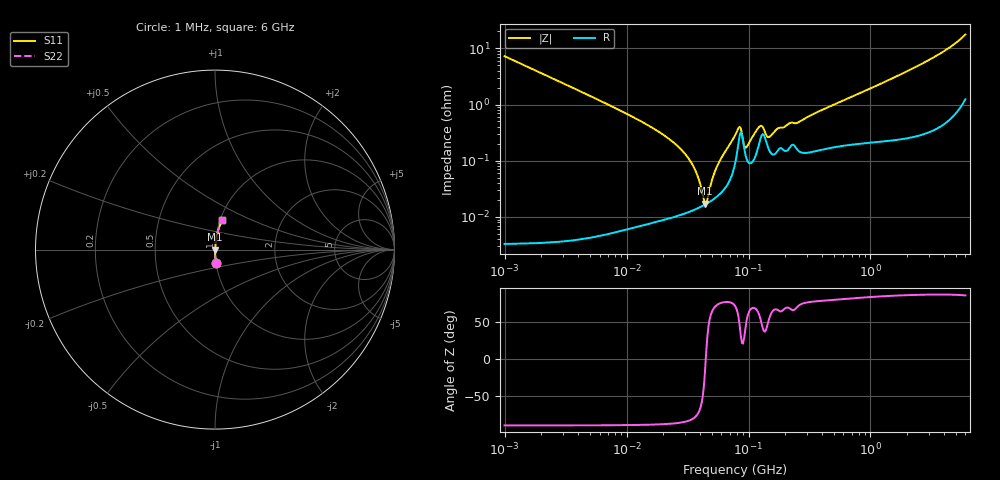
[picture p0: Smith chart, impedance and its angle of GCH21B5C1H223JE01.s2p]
!Murata Part Number: GCH21B5C1H223JE01
!These Parameters are Measured in Series Mode Connection
!Data Generated on Jun 19, 2026
!  o--ll--o
!Port1  Port2
!  o------o
!Operation Temp=25[degC], DC Bias Voltage=0[V]
!Freq. Start=1000[kHz] Stop=6[GHz] 401[Steps]
# Hz S RI R 50
!Freq.(Hz) S11(Real) S11(Imag) S21(Real) S21(Imag) S12(Real) S12(Imag) S22(Real) S22(Imag)
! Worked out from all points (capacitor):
!   401 points, 1 MHz to 6 GHz, reference 50 ohm
!   read as one part in series: C = 22 nF near 1.044 MHz
!   lowest |Z| = 17.3 mohm at 44 MHz (marker M1)
!   series resonance near 44.62 MHz, so ESL is about 580 pH
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1000000  0.00523 -0.0719  0.9948 0.0719  0.9948 0.0719  0.00523 -0.0719
4293785  0.000318 -0.0167  0.9997 0.0167  0.9997 0.0167  0.000318 -0.0167
1.843659e7  9.47e-05 -0.00326  0.9999 0.00326  0.9999 0.00326  9.47e-05 -0.00326
2.554826e7  0.000106 -0.00192  0.9999 0.00192  0.9999 0.00192  0.000106 -0.00192
3.245342e7  0.000124 -0.00107  0.9999 0.00107  0.9999 0.00107  0.000124 -0.00107
3.779011e7  0.000141 -0.000556  0.9999 0.000556  0.9999 0.000556  0.000141 -0.000556
4.400437e7  0.000166 -4.69e-05  0.9998 4.69e-05  0.9998 4.69e-05  0.000166 -4.69e-05
4.596069e7  0.000176 0.000101  0.9998 -0.000101  0.9998 -0.000101  0.000176 0.000101
5.124051e7  0.000205 0.000483  0.9998 -0.000483  0.9998 -0.000483  0.000205 0.000483
5.589783e7  0.000238 0.000809  0.9998 -0.000809  0.9998 -0.000809  0.000238 0.000809
7.745967e7  0.000888 0.00268  0.9991 -0.00268  0.9991 -0.00268  0.000888 0.00268
8.450008e7  0.00279 0.00286  0.9972 -0.00286  0.9972 -0.00286  0.00279 0.00286
9.218041e7  0.00163 0.000892  0.9984 -0.000892  0.9984 -0.000892  0.00163 0.000892
9.627852e7  0.00109 0.00136  0.9989 -0.00136  0.9989 -0.00136  0.00109 0.00136
1.249896e8  0.00242 0.00339  0.9976 -0.00339  0.9976 -0.00339  0.00242 0.00339
1.487431e8  0.00149 0.00221  0.9985 -0.00221  0.9985 -0.00221  0.00149 0.00221
1.770109e8  0.00161 0.00347  0.9984 -0.00347  0.9984 -0.00347  0.00161 0.00347
2.561955e8  0.00152 0.00457  0.9985 -0.00457  0.9985 -0.00457  0.00152 0.00457
3.325952e8  0.00147 0.00644  0.9985 -0.00644  0.9985 -0.00644  0.00147 0.00644
1.428092e9  0.003 0.0273  0.997 -0.0273  0.997 -0.0273  0.003 0.0273
3.483508e9  0.00904 0.0729  0.991 -0.0729  0.991 -0.0729  0.00904 0.0729
6e9  0.0411 0.1662  0.9589 -0.1662  0.9589 -0.1662  0.0411 0.1662
